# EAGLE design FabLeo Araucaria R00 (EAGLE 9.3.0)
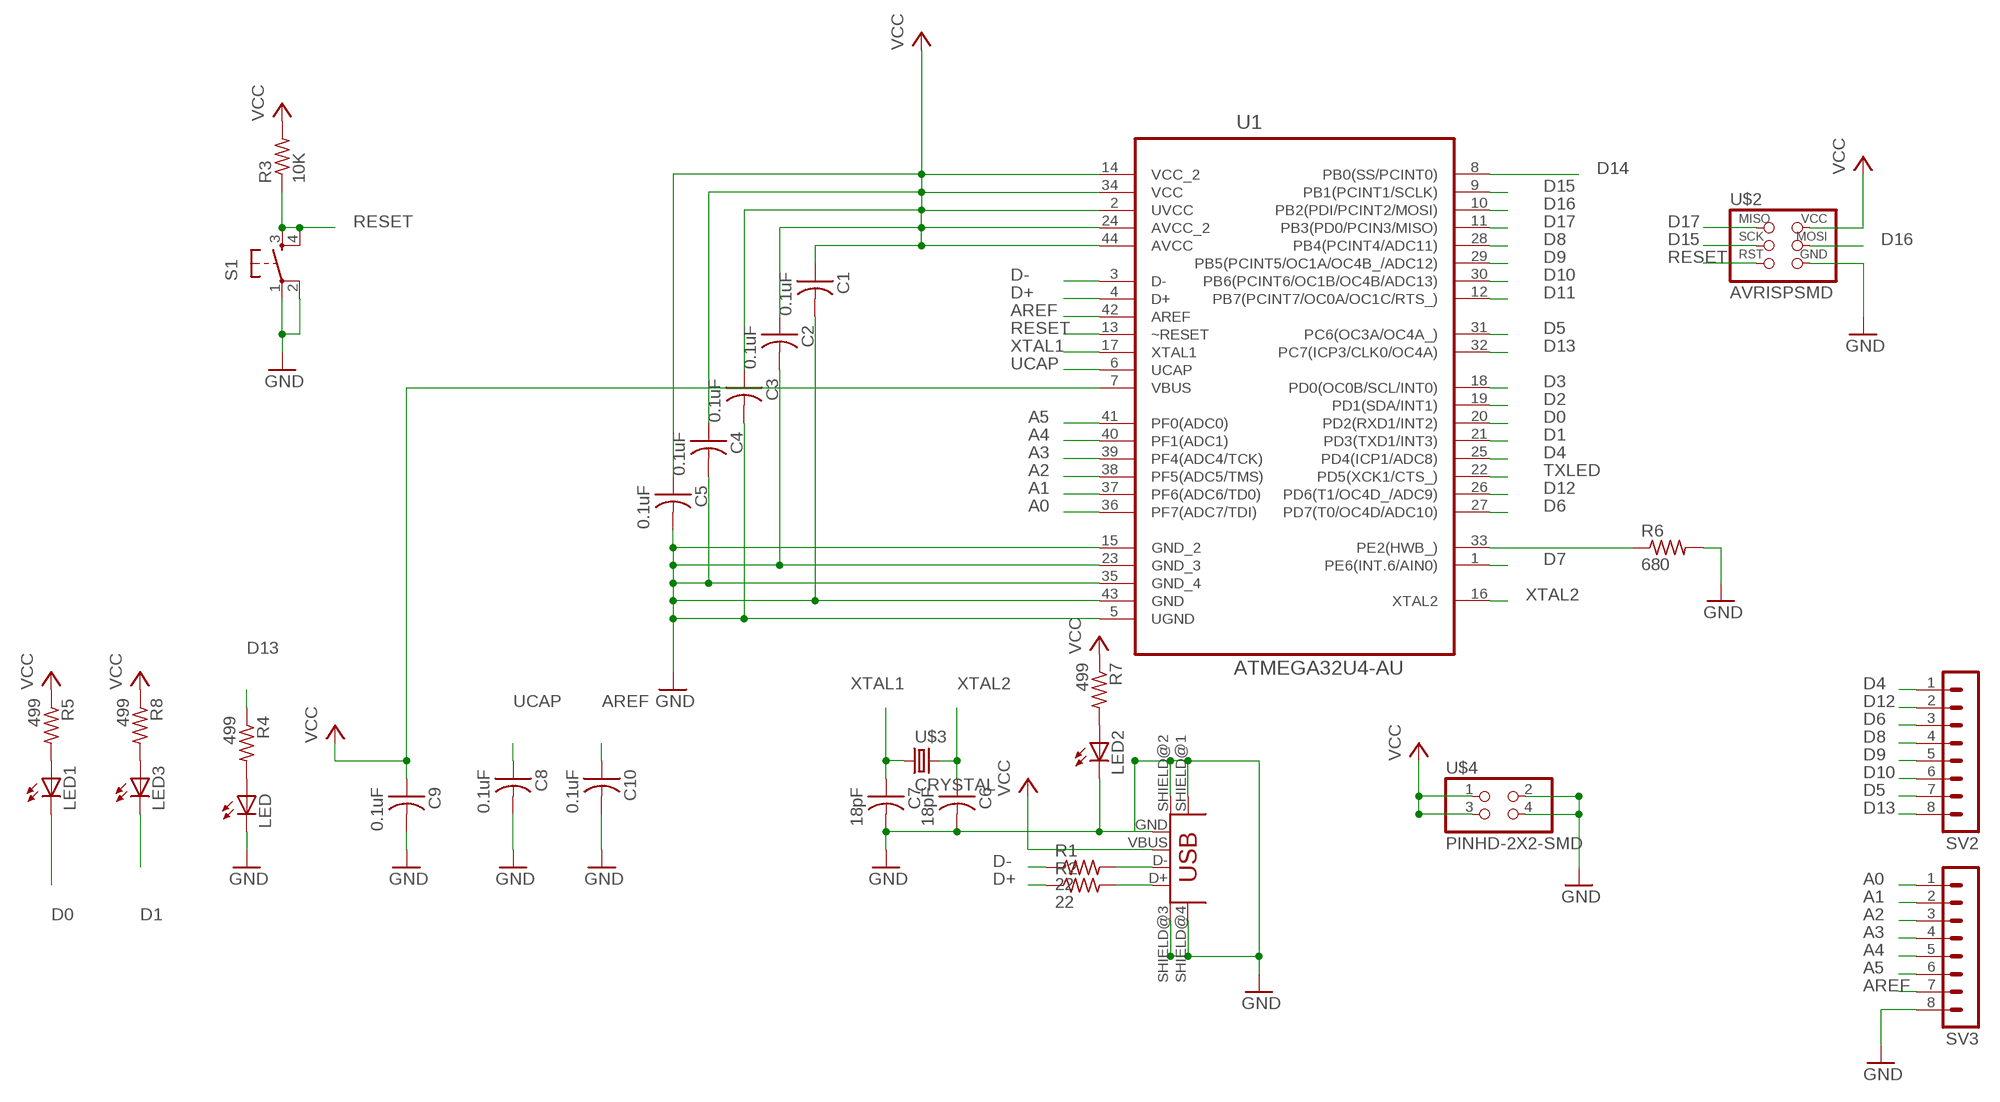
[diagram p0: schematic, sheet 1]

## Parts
C1  0.1uF  CAP-US1206FAB  [C1206FAB]
C2  0.1uF  CAP-US1206FAB  [C1206FAB]
C3  0.1uF  CAP-US1206FAB  [C1206FAB]
C4  0.1uF  CAP-US1206FAB  [C1206FAB]
C5  0.1uF  CAP-US1206FAB  [C1206FAB]
C6  18pF  CAP-US1206FAB  [C1206FAB]
C7  18pF  CAP-US1206FAB  [C1206FAB]
C8  0.1uF  CAP-US1206FAB  [C1206FAB]
C9  0.1uF  CAP-US1206FAB  [C1206FAB]
C10  0.1uF  CAP-US1206FAB  [C1206FAB]
LED  LED1206  [1206]
LED1  LED1206  [1206]
LED2  LED1206  [1206]
LED3  LED1206  [1206]
R1  22  RES-US1206FAB  [R1206FAB]
R2  22  RES-US1206FAB  [R1206FAB]
R3  10K  RES-US1206FAB  [R1206FAB]
R4  499  RESISTOR1206  [1206]
R5  499  RESISTOR1206  [1206]
R6  680  RES-US1206FAB  [R1206FAB]
R7  499  RESISTOR1206  [1206]
R8  499  RESISTOR1206  [1206]
S1  6MM_SWITCH6MM_SWITCH  [6MM_SWITCH]
SV2  MA08-1  [MA08-1]
SV3  MA08-1  [MA08-1]
U1  ATMEGA32U4-AU  [QFP80P1200X1200X120-44N]
U$1  USB_MINIB  [USB_MINIB]
U$2  AVRISPSMD  [2X03SMD]
U$3  CRYSTAL  [2-SMD-5X3MM]
U$4  PINHD-2X2-SMD  [2X02SMD]

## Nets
A0: SV3.1 U1.36(PF7(ADC7/TDI))
A1: SV3.2 U1.37(PF6(ADC6/TD0))
A2: SV3.3 U1.38(PF5(ADC5/TMS))
A3: SV3.4 U1.39(PF4(ADC4/TCK))
A4: SV3.5 U1.40(PF1(ADC1))
A5: SV3.6 U1.41(PF0(ADC0))
AREF: C10.1 SV3.7 U1.42(AREF)
D0: LED1.2(C) U1.20(PD2(RXD1/INT2))
D1: LED3.2(C) U1.21(PD3(TXD1/INT3))
D2: U1.19(PD1(SDA/INT1))
D3: U1.18(PD0(OC0B/SCL/INT0))
D4: SV2.1 U1.25(PD4(ICP1/ADC8))
D5: SV2.7 U1.31(PC6(OC3A/OC4A_))
D6: SV2.3 U1.27(PD7(T0/OC4D/ADC10))
D7: U1.1(PE6(INT.6/AIN0))
D8: SV2.4 U1.28(PB4(PCINT4/ADC11))
D9: SV2.5 U1.29(PB5(PCINT5/OC1A/OC4B_/ADC12))
D10: SV2.6 U1.30(PB6(PCINT6/OC1B/OC4B/ADC13))
D11: U1.12(PB7(PCINT7/OC0A/OC1C/RTS_))
D12: SV2.2 U1.26(PD6(T1/OC4D_/ADC9))
D13: R4.1 SV2.8 U1.32(PC7(ICP3/CLK0/OC4A))
D14: U1.8(PB0(SS/PCINT0))
D15: U1.9(PB1(PCINT1/SCLK)) U$2.3(SCK)
D16: U1.10(PB2(PDI/PCINT2/MOSI)) U$2.4(MOSI)
D17: U1.11(PB3(PD0/PCIN3/MISO)) U$2.1(MISO)
D+: R2.1 U1.4(D+)
D-: R1.1 U1.3(D-)
GND: C1.2 C2.2 C3.2 C4.2 C5.2 C6.2 C7.2 C8.2 C9.2 C10.2 LED2.2(C) LED.2(C) R6.2 S1.1(P) S1.2(P1) SV3.8 U1.5(UGND) U1.15(GND_2) U1.23(GND_3) U1.35(GND_4) U1.43(GND) U$1.GND U$1.SHIELD@1(SHIELD) U$1.SHIELD@2(SHIELD1) U$1.SHIELD@3(SHIELD2) U$1.SHIELD@4(SHIELD3) U$2.6(GND) U$4.2 U$4.4
N$1: R1.2 U$1.D-
N$2: R2.2 U$1.D+
N$3: LED.1(A) R4.2
N$4: LED1.1(A) R5.2
N$5: LED2.1(A) R7.2
N$6: LED3.1(A) R8.2
N$35: R6.1 U1.33(PE2(HWB_))
RESET: R3.1 S1.3(S) S1.4(S1) U1.13(~RESET) U$2.5(RST)
TXLED: U1.22(PD5(XCK1/CTS_))
UCAP: C8.1 U1.6(UCAP)
VCC: C1.1 C2.1 C3.1 C4.1 C5.1 C9.1 R3.2 R5.1 R7.1 R8.1 U1.2(UVCC) U1.7(VBUS) U1.14(VCC_2) U1.24(AVCC_2) U1.34(VCC) U1.44(AVCC) U$1.VBUS U$2.2(VCC) U$4.1 U$4.3
XTAL1: C7.1 U1.17(XTAL1) U$3.P$1
XTAL2: C6.1 U1.16(XTAL2) U$3.P$2

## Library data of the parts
C1-C10 = fab:CAP-US
LED LED1-LED3 = ng:LED
R1-R3 R6 = fab:RES-US: Resistor (US Symbol)
R4 R5 R7 R8 = ng:RESISTOR
S1 = ng:6MM_SWITCH: OMRON SWITCH
SV2 SV3 = con-lstb:MA08-1: PIN HEADER
U1 = Atmel_By_element14_Batch_1:ATMEGA32U4-AU: 8-bit Microcontroller with ISP Flash and USB Controller; MPN: ATMEGA32U4-AU; OC_FARNELL: 1748525; OC_NEWARK: 26R5633; PACKAGE: TQFP-44; SUPPLIER: Atmel
U$1 = fab:USB_MINIB
U$2 = fab:AVRISP
U$3 = fab:CRYSTAL
U$4 = fab:PINHD-2X2-SMD

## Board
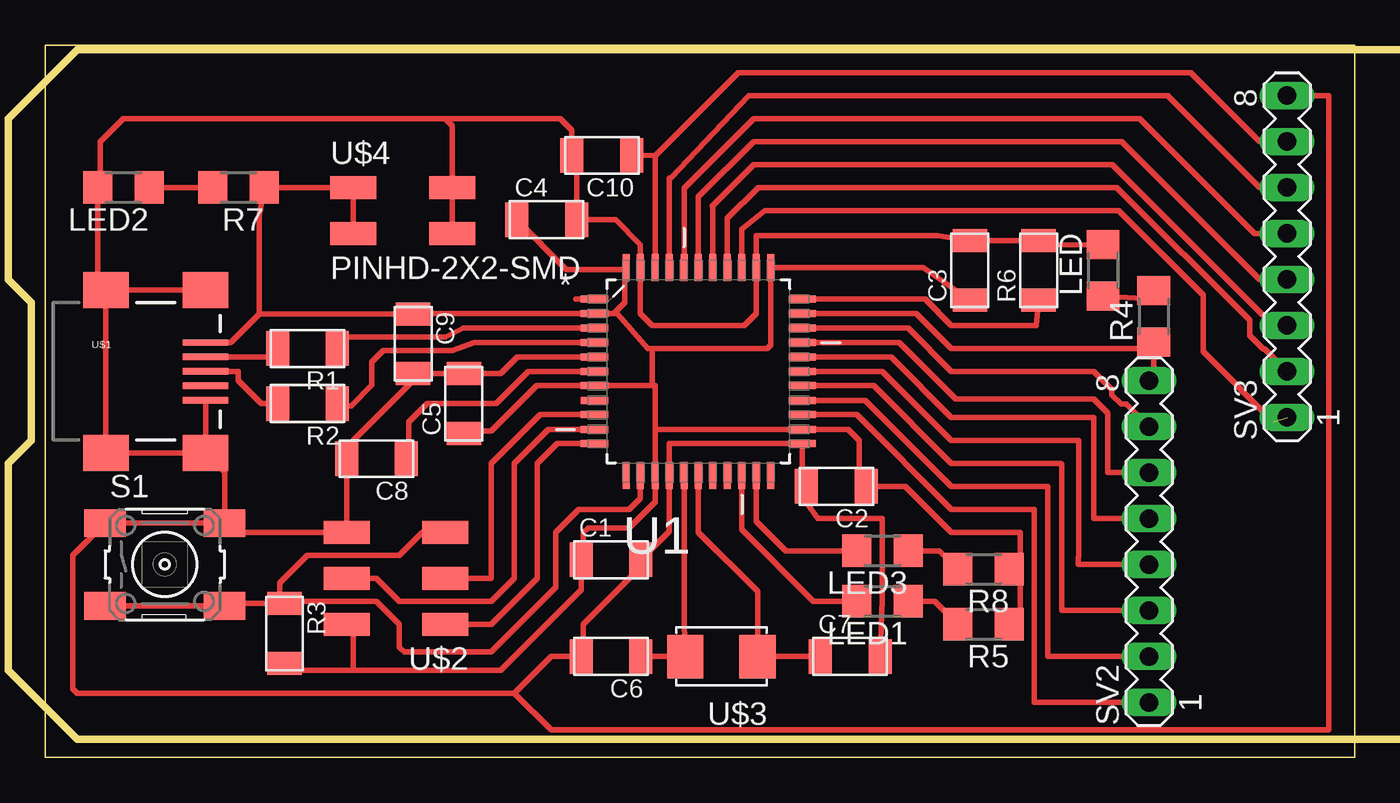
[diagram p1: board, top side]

Size 72.31 x 39.36 mm. Coordinates in mm from the lower left corner, seen from the top.
Outline: 0,0 72.31,0 72.31,39.36 0,39.36 0,0
Copper layers (1*16): Top 0.035mm / dielectric 1.5mm / Bottom 0.035mm
Design rules "default *": minimum track width 10mil, minimum drill 24mil, track to track 0.4mm, track to pad 0.4mm, pad to pad 0.4mm, via to via 0.4mm, smd to smd 0.4mm, copper to edge 40mil, drill to drill 0.4mm, minimum pad ring 10mil, minimum via ring 8mil, stop-mask expansion 4mil, vias tented up to drill 0mil, thermal gap 10mil
Milling: area -2,1 to 98.3,39.1

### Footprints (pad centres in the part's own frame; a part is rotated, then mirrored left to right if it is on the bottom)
C1206FAB = smd 1.27 x 1.905: 1 -1.651,0; 2 1.651,0
1206 = smd 1.6 x 1.803: 1 -1.422,0; 2 1.422,0
R1206FAB = smd 1.27 x 1.905: 1 -1.651,0; 2 1.651,0
6MM_SWITCH = smd 2.286 x 1.524: 1 -3.302,2.286; 2 3.302,2.286; 3 -3.302,-2.286; 4 3.302,-2.286
MA08-1 = drill 1.016 long: 1 -8.89,0; 2 -6.35,0; 3 -3.81,0; 4 -1.27,0; 5 1.27,0; 6 3.81,0; 7 6.35,0; 8 8.89,0
QFP80P1200X1200X120-44N = smd 1.5 x 0.38: 1 -5.74,3.988; 2 -5.74,3.2; 3 -5.74,2.388; 4 -5.74,1.6; 5 -5.74,0.787; 6 -5.74,0; 7 -5.74,-0.787; 8 -5.74,-1.6; 9 -5.74,-2.388; 10 -5.74,-3.2; 11 -5.74,-3.988; 23 5.74,-3.988; 24 5.74,-3.2; 25 5.74,-2.388; 26 5.74,-1.6; 27 5.74,-0.787; 28 5.74,0; 29 5.74,0.787; 30 5.74,1.6; 31 5.74,2.388; 32 5.74,3.2; 33 5.74,3.988 | smd 0.38 x 1.5: 12 -3.988,-5.74; 13 -3.2,-5.74; 14 -2.388,-5.74; 15 -1.6,-5.74; 16 -0.787,-5.74; 17 0,-5.74; 18 0.787,-5.74; 19 1.6,-5.74; 20 2.388,-5.74; 21 3.2,-5.74; 22 3.988,-5.74; 34 3.988,5.74; 35 3.2,5.74; 36 2.388,5.74; 37 1.6,5.74; 38 0.787,5.74; 39 0,5.74; 40 -0.787,5.74; 41 -1.6,5.74; 42 -2.388,5.74; 43 -3.2,5.74; 44 -3.988,5.74
USB_MINIB = smd 2.5 x 0.35: D+ 3.77,0; D- 3.77,0.8; GND 3.77,-1.6; ID 3.77,-0.8; VBUS 3.77,1.6 | smd 2.5 x 2: SHIELD@1 -1.73,-4.5; SHIELD@2 -1.73,4.5; SHIELD@3 3.77,4.5; SHIELD@4 3.77,-4.5
2X03SMD = smd 2.54 x 1.27: 1 -2.54,2.54; 2 2.92,2.54; 3 -2.54,0; 4 2.92,0; 5 -2.54,-2.54; 6 2.92,-2.54
2-SMD-5X3MM = smd 2 x 2.4: P$1 -2,0; P$2 2,0
2X02SMD = smd 2.54 x 1.27: 1 -2.54,1.27; 2 2.92,1.27; 3 -2.54,-1.27; 4 2.92,-1.27

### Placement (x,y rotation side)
C1  31.24,10.92 0 top
C2  43.69,14.99 180 top
C3  51.05,26.92 90 top
C4  27.69,29.72 0 top
C5  23.11,19.56 90 top
C6  31.24,5.59 180 top
C7  44.45,5.59 0 top
C8  18.29,16.51 180 top
C9  20.32,22.86 270 top
C10  30.73,33.27 180 top
LED  58.42,26.92 90 top
LED1  46.23,8.64 180 top
LED2  4.32,31.5 180 top
LED3  46.23,11.43 180 top
R1  14.48,22.61 180 top
R2  14.48,19.56 180 top
R3  13.21,6.86 270 top
R4  61.21,24.38 90 top
R5  51.82,7.37 180 top
R6  54.86,26.92 90 top
R7  10.67,31.5 180 top
R8  51.82,10.41 180 top
S1  6.6,10.67 0 top
SV2  60.96,11.94 90 top
SV3  68.58,27.69 90 top
U1  36.07,21.34 0 top
U$1  5.08,21.34 0 top
U$2  19.56,9.91 180 top
U$3  37.34,5.59 180 top
U$4  19.56,30.23 0 top

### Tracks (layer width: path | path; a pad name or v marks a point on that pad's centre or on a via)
A0  (1 unrouted)
  Top 0.305: U1.36 38.46,29.21 39.73,30.23 59.28,30.23 63.94,25.57 63.94,22.42 67.82,18.54
A1
  Top 0.305: U1.37 37.67,29.79 39.37,31.5 59.18,31.5 66.5,24.17 66.5,23.33 67.27,22.56 67.35,22.56 SV3.2
A2
  Top 0.305: U1.38 36.86,30.48 36.83,30.48 39.12,32.77 58.93,32.77 67.82,23.88 SV3.3
A3
  Top 0.305: U1.39 36.07,30.99 39.12,34.04 59.44,34.04 67.06,26.42 SV3.4
A4
  Top 0.305: U1.40 35.28,31.5 35.31,31.5 39.12,35.31 60.45,35.31 66.8,28.96 SV3.5
A5
  Top 0.305: U1.41 34.47,32 34.54,32 38.86,36.58 61.98,36.58 67.06,31.5 SV3.6
AREF
  Top 0.305: 33.68,33.25 C10.1 | 33.68,33.25 38.28,37.85 63.25,37.85 67.06,34.04 SV3.7 | 33.68,33.25 U1.42
D0
  Top 0.305: U1.20 38.46,12.6 42.42,8.64 LED1.2
D1
  Top 0.305: U1.21 39.27,13.06 40.89,11.43 LED3.2
D4
  Top 0.305: U1.25 44.81,18.95 50.04,13.72 54.59,13.72 54.61,13.7 54.61,3.05 SV2.1
D5
  Top 0.305: U1.31 47.65,23.72 50.04,21.34 57.91,21.34 58.91,20.34 58.91,20.04 59.41,19.54 59.71,19.54 SV2.7
D6
  Top 0.305: U1.27 45.75,20.55 50.04,16.26 56.08,16.26 56.13,16.2 56.13,8.13 SV2.3
D7
  Top 0.305: U1.1 29.29,25.32
D8
  Top 0.305: U1.28 46.23,21.34 50.04,17.53 57.08,17.53 57.08,11.1 57.04,11.07 57.04,10.67 SV2.4
D9
  Top 0.305: U1.29 46.71,22.12 50.04,18.8 57.91,18.8 57.91,13.21 SV2.5
D10
  Top 0.305: U1.30 47.17,22.94 50.29,19.81 57.91,19.81 58.67,19.05 58.67,15.75 SV2.6
D12
  Top 0.305: U1.26 45.29,19.74 50.04,14.99 55.37,14.99 55.37,5.59 SV2.2
D13
  Top 0.305: U1.32 48.11,24.54 50.04,22.61 60.86,22.61 R4.1 | R4.1 61.37,22.96 | SV2.8 61.21,20.83 | 61.21,20.83 62.13,20.83 | R4.1 61.21,20.83
D15
  Top 0.305: U1.9 27.33,18.95 24.64,16.26 24.64,9.91 U$2.3
D16
  Top 0.305: U1.10 27.79,18.14 25.91,16.26 25.91,9.91 24.64,8.64 19.56,8.64 18.29,9.91 U$2.4
D17
  Top 0.305: U1.11 28.27,17.35 27.18,16.26 27.18,9.91 24.64,7.37 U$2.1
D+
  Top 0.305: U1.4 23.7,22.94 22.48,22.48 18.67,22.48 18.03,21.84 18.03,20.57 16.89,19.43 16.26,19.43 R2.1
D-
  Top 0.305: U1.3 23.09,23.72 22.1,23.24 16.26,23.24 16,22.73 R1.1
GND
  Top 0.305: U$1.GND U$1.SHIELD@4 | S1.2 S1.1 1.52,11.18 1.52,3.81 1.78,3.56 25.91,3.56 | U$1.SHIELD@4 U$1.SHIELD@1 U$1.SHIELD@2 | 8.89,25.84 U$1.SHIELD@3 U$1.SHIELD@2 | U1.5 26.06,22.12 25.15,21.21 C5.2 C9.2 20.32,20.83 17.02,17.53 17.02,16.89 C8.2 U$2.6 9.91,12.45 S1.2 | U$1.SHIELD@2 2.9,25.84 LED2.2 3.05,31.65 3.05,34.04 4.32,35.31 22.1,35.31 | LED.2 55.86,28.32 R6.2 C3.2 49.25,28.85 39.27,28.85 U1.35 39.27,24.54 38.61,23.88 33.53,23.88 32.87,24.54 U1.43 32.87,28.35 31.5,29.72 C4.2 29.34,33.02 C10.2 29.08,34.67 28.45,35.31 22.1,35.31 | C7.2 46.23,8.76 46.23,13.21 42.67,13.21 42.04,14.1 C2.2 41.81,15.21 U1.23 34.47,17.35 U1.15 34.47,12.5 C1.2 32.89,10.54 29.72,7.37 29.72,5.71 C6.2 27.94,5.59 25.91,3.56 | U$4.2 U$4.4 22.48,34.93 22.1,35.31 | U$1.SHIELD@4 9.91,15.78 S1.2 | 25.91,3.56 27.94,1.52 70.87,1.52 70.87,36.58 SV3.8
N$1
  Top 0.305: U$1.D- 12.83,22.14 R1.2
N$2
  Top 0.305: R2.2 11.94,19.56 10.67,20.83 10.67,21.34 U$1.D+
N$3
  Top 0.305: R4.2 60.65,25.36 LED.1
N$4
  Top 0.305: LED1.1 49.12,8.64 R5.2
N$5
  Top 0.305: R7.2 LED2.1
N$6
  Top 0.305: LED3.1 49.38,11.43 R8.2
N$35
  Top 0.305: U1.33 48.59,25.32 50.04,23.88 54.74,23.88 R6.1
RESET
  Top 0.305: S1.3 S1.4 9.91,8.51 R3.1 | U1.13 32.87,14.33 32.26,13.72 29.46,13.72 28.19,12.45 28.19,9.4 24.64,5.84 19.81,5.84 19.56,6.1 19.56,7.37 18.29,8.64 13.34,8.64 R3.1 | U$2.5 20.83,12.45 19.56,11.18 14.48,11.18 12.95,9.65 12.95,8.76 R3.1
UCAP
  Top 0.305: U1.6 26.67,21.34 24.89,19.56 21.08,19.56 20.07,18.54 20.07,16.64 C8.1
VCC
  Top 0.305: U1.2 31.39,24.54 32,25.15 32,27 U1.44 31.83,26.97 28.78,26.97 C4.1 26.16,29.59 | 40.13,27 U1.34 | U1.2 20.35,24.54 C9.1 11.81,24.51 | 11.81,24.51 10.24,22.94 U$1.VBUS | 11.81,24.51 11.81,29.95 R7.1 U$4.1 U$4.3 | U1.34 48.49,27.08 C3.1 | 53.85,10.06 53.85,12.45 50.04,12.45 47.5,14.99 C2.1 44.96,15.37 44.96,17.53 44.35,18.14 U1.24 33.68,18.14 | 53.85,10.06 R8.1 | 52.58,7.37 R5.1 53.85,7.37 53.85,10.06 | 17.02,4.83 13.59,4.83 R3.2 | U$2.2 17.02,7.37 17.02,4.83 | U1.2 31.6,24.54 33.27,22.61 33.53,22.61 | 17.02,4.83 25.15,4.83 29.59,9.27 C1.1 29.72,11.05 29.72,12.45 29.97,12.7 32.26,12.7 33.68,14.12 U1.14 33.68,18.14 | U1.34 40.06,22.78 39.88,22.61 33.53,22.61 | 33.53,20.55 U1.7 27.15,20.55 24.64,18.03 22.73,18.03 C5.1 | 33.53,20.55 33.68,20.55 33.68,18.14 | 33.53,22.61 33.53,20.55
XTAL1
  Top 0.305: C7.1 U$3.P$1 39.34,9.18 36.07,12.45 U1.17
XTAL2
  Top 0.305: C6.1 U$3.P$2 35.28,7.42 U1.16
